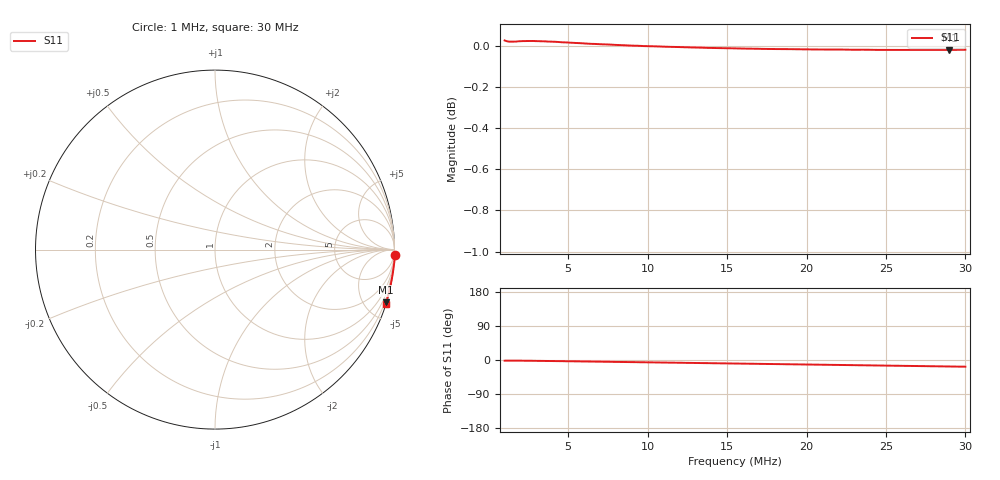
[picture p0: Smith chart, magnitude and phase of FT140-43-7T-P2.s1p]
! ListType=Log
!!FT140-43 7T Port 2
# MHz S DB R 50
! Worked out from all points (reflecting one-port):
!   101 points, 1 MHz to 30 MHz, reference 50 ohm
!   lowest |S11| = 0.0 dB at 29 MHz (marker M1), VSWR 874.09, Z = 2.58 - j332 ohm
!   phase of S11 starts at -2 deg and turns -16 deg over the sweep
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1  0.03 -1.9
1.107423  0.02 -1.8
1.226386  0.02 -1.7
1.358129  0.02 -1.7
1.504023  0.02 -1.7
1.609893  0.02 -1.7
1.782833  0.02 -1.7
1.908328  0.02 -1.8
2.113327  0.02 -1.8
2.505087  0.02 -2.0
3.072204  0.02 -2.3
3.767708  0.02 -2.6
4.780527  0.02 -3.2
6.065607  0.01 -3.9
8.52288  0.00 -5.3
10.45234  -0.00 -6.4
11.97563  -0.01 -7.3
13.2621  -0.01 -8.0
15.72057  -0.01 -9.4
16.82715  -0.01 -10.1
19.27949  -0.02 -11.5
22.08922  -0.02 -13.1
22.85344  -0.02 -13.5
23.6441  -0.02 -14.0
25.30843  -0.02 -15.0
27.08991  -0.02 -16.0
28.9968  -0.02 -17.1
30  -0.02 -17.7
